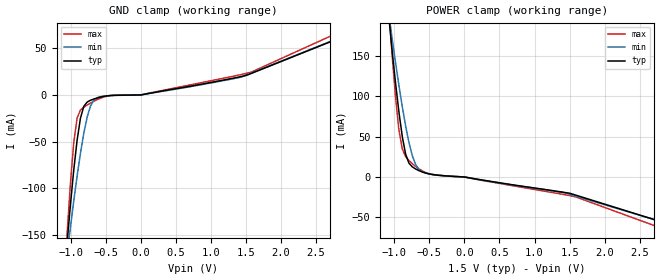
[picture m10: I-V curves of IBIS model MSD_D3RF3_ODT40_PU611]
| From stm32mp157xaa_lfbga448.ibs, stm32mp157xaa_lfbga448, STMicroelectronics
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[Model] MSD_D3RF3_ODT40_PU611
Model_type   Input
C_comp 2.332pF   2.290pF   2.410pF
Vinh = 925.000mV
Vinl = 575.000mV
[Temperature Range]   25.000   125.000   -40.000
[Voltage Range]   1.500V   1.425V   1.575V
[GND Clamp Reference]   0.00V   0.00V   0.00V
[POWER Clamp Reference]   1.500V   1.425V   1.575V
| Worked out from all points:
|   GND clamp passes 1 mA (typ) near -0.48 V on its own axis
|   POWER clamp passes 1 mA (typ) near -0.21 V on its own axis
[GND Clamp]
-1.48V    -589.9mA   -457.5mA   -789mA
-1.05V    -159.5mA   -171.8mA   -149.7mA
-1.002V   -118.1mA   -142.3mA   -95.22mA
-954.6mV  -80.67mA   -113.9mA   -51.24mA
-906.8mV  -48.74mA   -87.17mA   -24.9mA
-859.1mV  -25.02mA   -62.71mA   -16.2mA
-763.6mV  -7.648mA   -23.89mA   -10.82mA
-715.9mV  -5.7mA     -11.92mA   -8.73mA
-620.5mV  -3.244mA   -2.964mA   -4.992mA
900nV     12.83nA    12.02nA    14.83nA
1.575V    23.03mA    23.49mA    24.42mA
2.959V    64.73mA    65.07mA    71.75mA
[Power Clamp]
-1.459V   583.5mA    459.2mA    772.8mA
-1.077V   198mA      201.6mA    208.4mA
-1.03V    155.5mA    171.2mA    150.2mA
-981.8mV  116.3mA    141.7mA    98.43mA
-934.1mV  80.59mA    113.5mA    58.16mA
-886.4mV  50.22mA    87.28mA    34.9mA
-838.6mV  28.34mA    63.46mA    25.32mA
-790.9mV  17.15mA    42.82mA    20.44mA
-695.5mV  9.9mA      15.3mA     13.1mA
-504.6mV  3.802mA    3.902mA    3.994mA
1.548V    -21.48mA   -22.72mA   -23.9mA
2.98V     -60.24mA   -59.98mA   -68.95mA
